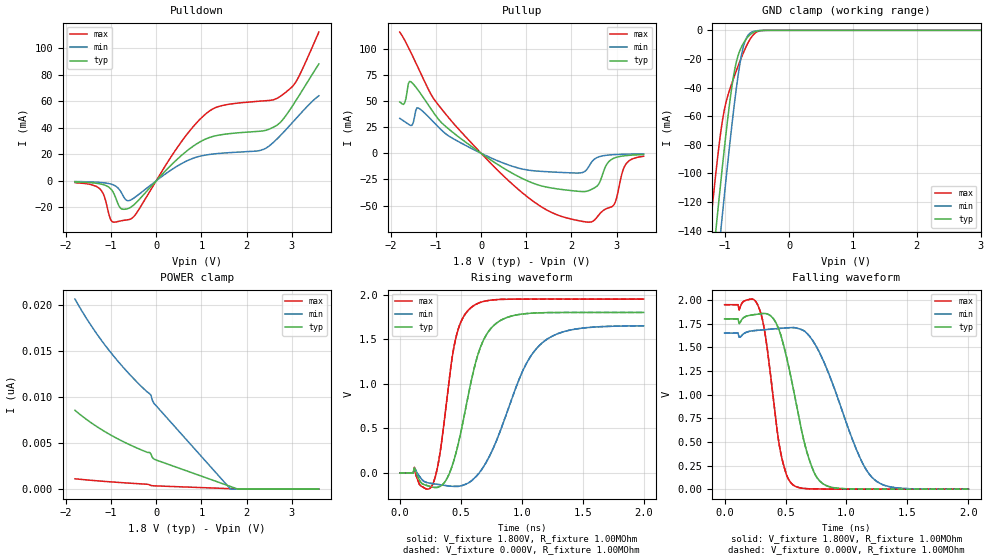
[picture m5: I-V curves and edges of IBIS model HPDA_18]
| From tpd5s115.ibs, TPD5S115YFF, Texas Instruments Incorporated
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[Model]   HPDA_18
Model_type   I/O
Vinl = 0.4V
Vinh = 1.0V
Vmeas = 1.500V
Vref = 0V
Cref =15pF
|   typ   min   max
|3-state
C_comp   1.6799pF   1.5123pF   1.9969pF
|pulldown
|C_comp   1.7226pF   1.5177pF   2.1617pF
|pullup
|C_comp   1.7546pF   1.5733pF   2.1821pF
[Voltage Range]   1.800V   1.650V   1.950V
|Junction temperature
[Temperature Range]   40.0   100.0   -40.0
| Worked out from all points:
|   slope of the pulldown table from 0 to 0.27 V, typ, clamps not added: 27.5 ohm
|   slope of the pullup table from 0 to 0.27 V, typ, clamps not added: 33.9 ohm
|   GND clamp passes 1 mA (typ) near -0.54 V on its own axis
|   falling waveform, V_fixture 1.800V, R_fixture 1.00MOhm: 20-80 % time 182ps typ, 288ps min, 118ps max; typ from 1.8 V to 0 V
|   rising waveform, V_fixture 1.800V, R_fixture 1.00MOhm: 20-80 % time 185ps typ, 296ps min, 121ps max; typ from 0 V to 1.8 V
|   rising waveform, V_fixture 0.000V, R_fixture 1.00MOhm: 20-80 % time 185ps typ, 296ps min, 121ps max; typ from 0 V to 1.8 V
|   falling waveform, V_fixture 0.000V, R_fixture 1.00MOhm: 20-80 % time 182ps typ, 288ps min, 118ps max; typ from 1.8 V to 0 V
|ambient temperature   25   85   -40|
[Pulldown]
|   Voltage   I(typ)   I(min)   I(max)
-1.8V     -880.8uA   -561.3uA   -1.419mA
-1.23V    -2.434mA   -1.3mA     -6.798mA
-958.8mV  -8.362mA   -2.998mA   -31.18mA
-796mV    -20.53mA   -7.635mA   -30.38mA
-551.8mV  -19.72mA   -14.3mA    -28.61mA
452.3mV   15.88mA    10.84mA    24.44mA
967.8mV   29.39mA    18.59mA    46.46mA
1.375V    34.4mA     20.61mA    56.02mA
2.325V    37.53mA    23.15mA    60.23mA
2.786V    45.56mA    35.5mA     64.73mA
3.112V    61.63mA    47.64mA    75.85mA
3.6V      88.25mA    64.21mA    112.3mA
[GND Clamp]
|   Voltage   I(typ)   I(min)   I(max)
-1.8V     -449.5mA   -485mA     -405.8mA
-1.23V    -178.5mA   -213.8mA   -136.1mA
-1.149V   -141.5mA   -176.4mA   -101.2mA
-1.122V   -129.4mA   -164.1mA   -90.34mA
-1.067V   -105.7mA   -139.7mA   -70.71mA
-985.9mV  -71.98mA   -104.1mA   -50.23mA
-850.3mV  -27.41mA   -49.61mA   -31.36mA
-768.8mV  -14.08mA   -23.4mA    -21.67mA
-714.6mV  -9.108mA   -11.41mA   -15.72mA
-578.9mV  -1.974mA   -1.135mA   -4.193mA
-361.8mV  -25.41uA   -18.7uA    -25.54uA
3.6V      0A         0A         0A
[Pullup]
|   Voltage   I(typ)   I(min)   I(max)
-1.8V     49.11mA    33.39mA    115.9mA
-1.691V   48.17mA    30.22mA    108.1mA
-1.556V   68.39mA    26.54mA    96.53mA
-1.393V   60.29mA    43.32mA    81.76mA
-633.2mV  20.24mA    14.37mA    29.7mA
642.2mV   -17.9mA    -11.7mA    -27.54mA
1.538V    -33.05mA   -17.82mA   -56.11mA
2.243V    -36.62mA   -18.44mA   -65.11mA
2.487V    -33.6mA    -6.467mA   -64.69mA
2.894V    -5.721mA   -1.449mA   -51.11mA
3.193V    -2.334mA   -883.3uA   -11.27mA
3.6V      -1.254mA   -571.4uA   -2.839mA
[POWER Clamp]
|   Voltage   I(typ)   I(min)   I(max)
-1.8V     8.578nA    20.68nA    1.128nA
-1.502V   7.432nA    18.24nA    989.7pA
-1.149V   6.293nA    15.76nA    846.9pA
-633.2mV  4.938nA    12.72nA    667.7pA
-226.1mV  4.061nA    10.69nA    542.2pA
-144.7mV  3.989nA    10.36nA    459pA
-117.6mV  3.825nA    10.23nA    397.8pA
-90.45mV  3.481nA    9.716nA    378.8pA
-36.18mV  3.243nA    9.248nA    362.2pA
1.646V    285.2pA    0A         54.23pA
1.809V    0A         0A         24.65pA
3.6V      0A         0A         0A
[Ramp]
R_load = 1.00MOhm
|   typ   min   max
dV/dt_r   1.080V/185.077ps 989.924mV/296.188ps   1.170V/121.020ps
dV/dt_f   1.080V/182.444ps 989.934mV/288.281ps   1.170V/117.716ps
[Falling Waveform]
V_fixture = 1.800V
V_fixture_min = 1.650V
V_fixture_max = 1.950V
R_fixture = 1.00MOhm
|   Time   V(typ)   V(min)   V(max)
0s        1.8V       1.65V      1.95V
280ps     1.852V     1.681V     1.924V
340ps     1.856V     1.687V     1.578V
460ps     1.633V     1.7V       387.5mV
560ps     1.086V     1.708V     47.01mV
690ps     329.9mV    1.628V     4.05mV
810ps     54.31mV    1.359V     1.197mV
1.08ns    1.442mV    422.6mV    285.5uV
1.22ns    617.3uV    111.3mV    177uV
2ns       61.91uV    83.49uV    44.64uV
[Rising Waveform]
V_fixture = 1.800V
V_fixture_min = 1.650V
V_fixture_max = 1.950V
R_fixture = 1.00MOhm
|   Time   V(typ)   V(min)   V(max)
0s        61.91uV    83.49uV    44.64uV
120ps     57.7mV     53.92mV    62.93mV
270ps     -158.3mV   -118.6mV   -126.7mV
330ps     -150.2mV   -130.6mV   223.3mV
460ps     218.8mV    -149.5mV   1.514V
600ps     1.116V     -73.07mV   1.871V
780ps     1.666V     320.4mV    1.943V
1.01ns    1.784V     1.151V     1.95V
1.16ns    1.797V     1.449V     1.95V
2ns       1.8V       1.65V      1.95V
[Rising Waveform]
V_fixture = 0.000V
V_fixture_min = 0.000V
V_fixture_max = 0.000V
R_fixture = 1.00MOhm
|   Time   V(typ)   V(min)   V(max)
0s        14.57uV    21.63uV    10.99uV
120ps     57.65mV    53.86mV    62.9mV
270ps     -158.5mV   -118.7mV   -126.8mV
330ps     -150.4mV   -130.8mV   223.1mV
460ps     218.5mV    -149.8mV   1.514V
600ps     1.116V     -73.46mV   1.871V
780ps     1.666V     320mV      1.943V
1.01ns    1.784V     1.15V      1.95V
1.16ns    1.797V     1.449V     1.95V
2ns       1.8V       1.65V      1.95V
[Falling Waveform]
V_fixture = 0.000V
V_fixture_min = 0.000V
V_fixture_max = 0.000V
R_fixture = 1.00MOhm
|   Time   V(typ)   V(min)   V(max)
0s        1.8V       1.65V      1.95V
280ps     1.852V     1.681V     1.924V
340ps     1.855V     1.687V     1.577V
460ps     1.633V     1.7V       387.4mV
560ps     1.086V     1.708V     46.96mV
690ps     329.8mV    1.628V     4.015mV
810ps     54.24mV    1.358V     1.163mV
1.08ns    1.394mV    422.4mV    251.8uV
1.22ns    569.4uV    111.2mV    143.3uV
2ns       14.57uV    21.63uV    10.99uV
